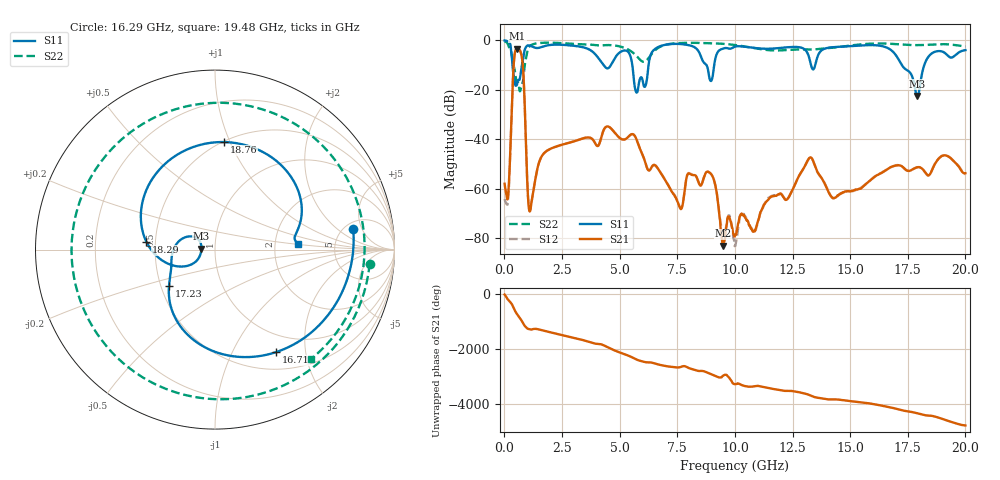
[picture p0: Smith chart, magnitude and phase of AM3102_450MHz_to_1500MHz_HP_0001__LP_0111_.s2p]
!Agilent Technologies,E8364B,MY43040894,A.07.50.67
!Agilent E8364B: A.07.50.67
!Date: Thursday, January 11, 2018 05:21:14
!Correction: S11(Full 2 Port(1,2))
!S21(Full 2 Port(1,2))
!S12(Full 2 Port(1,2))
!S22(Full 2 Port(1,2))
!S2P File: Measurements: S11, S21, S12, S22:
# Hz S  dB  R 50
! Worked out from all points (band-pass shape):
!   1601 points, 10 MHz to 20 GHz, reference 50 ohm
!   highest |S21| = -3.37 dB at 559.7 MHz (marker M1); lowest = -83.0 dB at 9.48 GHz (marker M2)
!   |S21| within 3 dB of the highest: 435.8 MHz to 749.4 MHz (313.6 MHz wide, 52.9 % of centre)
!   lowest |S11| = -22.4 dB at 17.91 GHz (marker M3), VSWR 1.16, Z = 43 + j0.413 ohm
!   |S11| at or under -10 dB: 350.4 MHz to 762.9 MHz (412.5 MHz wide, 74.1 % of centre); 5.55 GHz to 6.254 GHz (704.1 MHz wide, 11.9 % of centre); 17.24 GHz to 18.22 GHz (972.7 MHz wide, 5.49 % of centre)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
!   |S22| runs from -20.6 to -0.4 dB; largest |S21 - S12| = 0.0018
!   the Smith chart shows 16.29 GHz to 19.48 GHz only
!   S11 on the Smith chart (normalised r, x): 16.29 GHz: 6.01, +3.44; 16.71 GHz: 0.73, -1.50; 17.23 GHz: 0.55, -0.25; 18.29 GHz: 0.45, +0.04; 18.76 GHz: 0.51, +0.95; 19.48 GHz: 2.71, +0.20
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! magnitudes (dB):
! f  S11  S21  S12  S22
! 10 MHz  -0.1  -57.9  -64.1  -0.4
! 172.4 MHz  -0.6  -61.4  -63.3  -2.1
! 559.7 MHz  -17.2  -3.4  -3.4  -17.1
! 784.6 MHz  -8.9  -8.7  -8.7  -17.3
! 1.109 GHz  -2.2  -69.1  -68.8  -2.3
! 3.346 GHz  -2.7  -39.8  -39.8  -1.6
! 5.732 GHz  -21.1  -40.0  -40.0  -6.3
! 6.682 GHz  -2.7  -52.1  -52.0  -3.0
! 7.644 GHz  -1.5  -68.1  -67.5  -1.1
! 8.931 GHz  -16.2  -53.6  -53.7  -1.2
! 9.48 GHz  -3.4  -83.0  -78.0  -1.4
! 10.01 GHz  -2.5  -78.8  -82.9  -1.9
! 13.34 GHz  -11.1  -47.7  -47.7  -3.8
! 16.29 GHz  -2.2  -53.9  -53.8  -1.3
! 16.68 GHz  -3.3  -51.7  -51.7  -1.4
! 16.71 GHz  -3.5  -51.5  -51.5  -1.4
! 17.23 GHz  -9.8  -50.8  -50.8  -1.7
! 17.91 GHz  -22.4  -51.3  -51.3  -1.9
! 18.29 GHz  -8.3  -53.7  -53.8  -1.8
! 18.76 GHz  -4.4  -48.7  -48.6  -1.6
! 19.48 GHz  -6.7  -48.6  -48.6  -1.8
! 20 GHz  -4.0  -53.7  -54.1  -2.5
